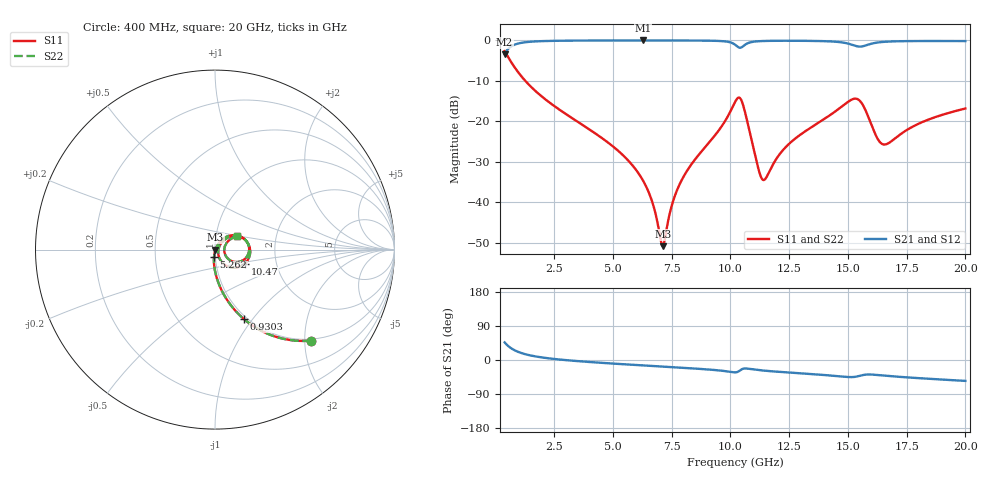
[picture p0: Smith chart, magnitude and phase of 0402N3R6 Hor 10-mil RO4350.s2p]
# GHz S MA R 50
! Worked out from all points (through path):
!   1960 points, 400 MHz to 20 GHz, reference 50 ohm
!   highest |S21| = -0.03 dB at 6.283 GHz (marker M1); lowest = -3.4 dB at 400 MHz (marker M2)
!   group delay of S21, straight-line fit = 9.69 ps
!   lowest |S11| = -50.9 dB at 7.123 GHz (marker M3), VSWR 1.01, Z = 50.3 - j0.0929 ohm
!   |S11| at or under -10 dB: 1.279 GHz to end of sweep
!   |S22| runs from -50.9 to -2.6 dB; largest |S21 - S12| = 0
!   S11 on the Smith chart (normalised r, x): 400 MHz: 0.96, -2.15; 930.3 MHz: 0.97, -0.91; 5.262 GHz: 0.99, -0.08; 10.47 GHz: 1.38, -0.22; 20 GHz: 1.26, +0.19
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0.4  0.7376 -43.4  0.6749 46.5  0.6749 46.5  0.7376 -43.4
0.9302705  0.421 -67.3  0.9062 22.6  0.9062 22.6  0.421 -67.3
1.79071  0.2258 -81.0  0.9729 8.7  0.9729 8.7  0.2258 -81.0
3.671669  0.09179 -92.6  0.9939 -3.7  0.9939 -3.7  0.09179 -92.6
5.262481  0.04234 -97.5  0.9967 -10.4  0.9967 -10.4  0.04234 -97.5
6.283002  0.01859 -96.6  0.9971 -14.3  0.9971 -14.3  0.01859 -96.6
6.663196  0.01044 -91.1  0.997 -15.7  0.997 -15.7  0.01044 -91.1
6.943338  0.004865 -72.2  0.9969 -16.7  0.9969 -16.7  0.004865 -72.2
7.12343  0.002861 -18.8  0.9968 -17.4  0.9968 -17.4  0.002861 -18.8
7.543645  0.009807 52.3  0.9965 -18.9  0.9965 -18.9  0.009807 52.3
7.923839  0.01854 58.6  0.996 -20.3  0.996 -20.3  0.01854 58.6
10.205  0.1738 19.6  0.8837 -32.6  0.8837 -32.6  0.1738 19.6
10.46514  0.1833 -25.3  0.8162 -25.3  0.8162 -25.3  0.1833 -25.3
11.20551  0.02525 -45.1  0.9756 -26.6  0.9756 -26.6  0.02525 -45.1
11.40562  0.0188 -10.0  0.9816 -27.9  0.9816 -27.9  0.0188 -10.0
12.30607  0.04624 45.3  0.9885 -32.2  0.9885 -32.2  0.04624 45.3
13.46667  0.08502 45.0  0.9842 -37.2  0.9842 -37.2  0.08502 45.0
15.35763  0.19 -2.2  0.8495 -43.9  0.8495 -43.9  0.19 -2.2
15.66779  0.1535 -25.9  0.8495 -39.4  0.8495 -39.4  0.1535 -25.9
16.32813  0.05697 -19.6  0.9457 -40.0  0.9457 -40.0  0.05697 -19.6
16.73834  0.0538 11.1  0.9662 -42.2  0.9662 -42.2  0.0538 11.1
20  0.1439 31.2  0.9797 -55.2  0.9797 -55.2  0.1439 31.2
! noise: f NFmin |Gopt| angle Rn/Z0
0.4  0.001246  0.7869  2.823  0.001202
2.571  0.00506  0.6782  6.973  0.003027
4.752  0.008132  0.6397  11.96  0.004216
6.933  0.01145  0.6309  16.94  0.005705
9.104  0.02133  0.7268  21.95  0.01497
11.29  0.03957  0.8106  27.27  0.04117
13.47  0.03203  0.7358  32.1  0.02242
15.64  0.1327  0.9192  37.27  0.3259
17.82  0.04163  0.7384  41.92  0.02786
20  0.03416  0.6634  46.19  0.01657
